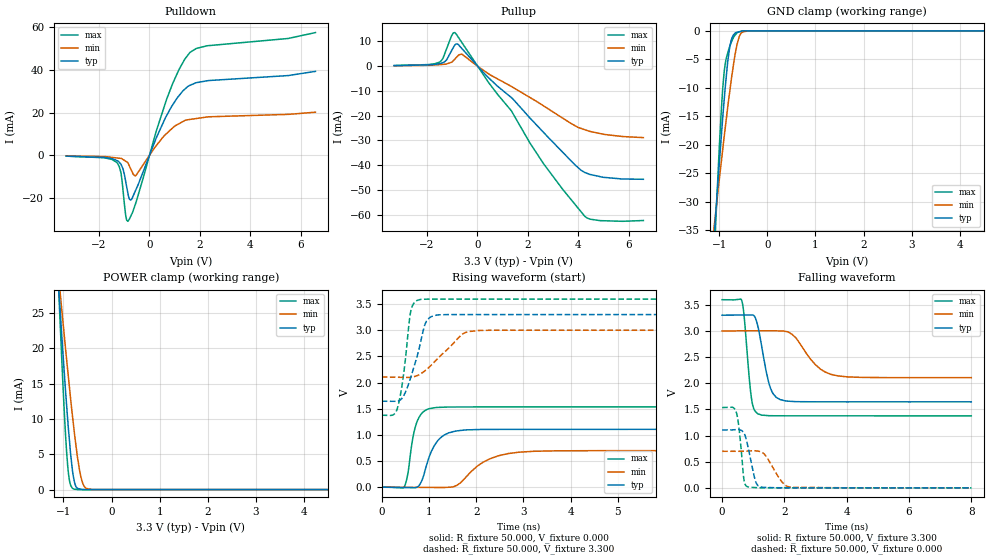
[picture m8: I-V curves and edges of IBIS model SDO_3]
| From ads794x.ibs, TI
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|   SDO 3.3V Model
[Model] SDO_3
Model_type   3-state
Polarity   Non-Inverting
Enable   Active-Low
Vmeas = 1.65
Vref = 1.65
Cref = 15pF
Rref = 50
|   typ   min   max
|   (Nom PVT)   (Fast PVT)  (Slow PVT)
|  (high input impedance)
C_comp   1.5797330e-12   1.2761490e-12   1.9045100e-12
|  (high output)
|C_comp   2.1280980e-12   1.7654750e-12   2.4622910e-12
|  (low output)
|C_comp   1.0558410e-12   8.2578200e-13   1.4524100e-12
[Voltage Range]   3.3   3   3.6
[Temperature Range]   27   125   -40
[Pullup Reference]   3.3   3   3.6
[Pulldown Reference]   0   0   0
[Power Clamp Reference]   3.3   3   3.6
[GND Clamp Reference]   0   0   0
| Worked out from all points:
|   slope of the pulldown table from 0 to 0.495 V, typ, clamps not added: 35.2 ohm
|   slope of the pullup table from 0 to 0.495 V, typ, clamps not added: 93 ohm
|   GND clamp passes 1 mA (typ) near -0.72 V on its own axis
|   POWER clamp passes 1 mA (typ) near -0.77 V on its own axis
|   falling waveform, R_fixture 50.000, V_fixture 3.300: 20-80 % time 325ps typ, 704ps min, 192ps max; typ from 3.3 V to 1.64 V
|   rising waveform, R_fixture 50.000, V_fixture 0.000: 20-80 % time 296ps typ, 612ps min, 176ps max; typ from 0 V to 1.11 V
|   rising waveform, R_fixture 50.000, V_fixture 3.300: 20-80 % time 302ps typ, 595ps min, 174ps max; typ from 1.64 V to 3.3 V
|   falling waveform, R_fixture 50.000, V_fixture 0.000: 20-80 % time 238ps typ, 426ps min, 149ps max; typ from 1.11 V to 0 V
[Pulldown]
|   Voltage   I(typ)   I(min)   I(max)
-3.3V     -352.2uA   -233.3uA   -375.8uA
-1.293V   -2.417mA   -1.214mA   -3.331mA
-1.135V   -4.022mA   -1.435mA   -7.896mA
-947mV    -11.94mA   -2.7mA     -27.63mA
-859.1mV  -17.48mA   -3.397mA   -30.89mA
-747.5mV  -20.98mA   -6.21mA    -28.68mA
-544.8mV  -16.32mA   -9.497mA   -22.46mA
688.3mV   18.76mA    10.3mA     26.47mA
1.169V    27.89mA    14.8mA     40.07mA
1.596V    32.73mA    16.8mA     48.04mA
2.285V    34.93mA    17.97mA    51.32mA
6.59V     39.34mA    20.22mA    57.52mA
[GND Clamp]
|   Voltage   I(typ)   I(min)   I(max)
-3.3V     -328.8mA   -220.3mA   -502.7mA
-1.091V   -34.15mA   -33.2mA    -37.08mA
-1.069V   -31.46mA   -31.46mA   -32.81mA
-962.1mV  -19.04mA   -23.34mA   -14.63mA
-925.9mV  -15mA      -20.65mA   -9.896mA
-894.4mV  -11.8mA    -18.35mA   -6.959mA
-790mV    -3.26mA    -11.15mA   -2.902mA
-733mV    -1.183mA   -7.554mA   -1.68mA
-658.6mV  -306.6uA   -3.608mA   -629.6uA
-552.4mV  -101.2uA   -492.2uA   -91.33uA
-387.7mV  -8.397uA   -5.302uA   -27.14uA
6.59V     0A         0A         0A
[Pullup]
|   Voltage   I(typ)   I(min)   I(max)
-3.3V     186uA      133.8uA    217.3uA
-1.51V    980uA      572.5uA    1.547mA
-1.223V   2.485mA    849.4uA    6.91mA
-1.022V   6.221mA    1.561mA    12.26mA
-894.4mV  8.451mA    2.812mA    13.54mA
-602.7mV  6.957mA    4.705mA    9.331mA
437mV     -4.631mA   -3.064mA   -6.524mA
1.346V    -12.7mA    -8.209mA   -18.02mA
2.658V    -27.13mA   -16.28mA   -39.88mA
4.258V    -42.95mA   -25.69mA   -60.62mA
4.872V    -44.67mA   -27.26mA   -62.45mA
6.59V     -45.74mA   -28.9mA    -62.4mA
[POWER Clamp]
|   Voltage   I(typ)   I(min)   I(max)
-3.3V     294.5mA    213.9mA    419.3mA
-1.091V   27.74mA    29.53mA    27.09mA
-1.06V    24.48mA    27.26mA    22.29mA
-970.1mV  15.31mA    20.9mA     9.4mA
-911.7mV  9.92mA     16.9mA     3.379mA
-859.1mV  5.671mA    13.4mA     812.3uA
-778.4mV  1.317mA    8.386mA    59.57uA
-708.3mV  165.6uA    4.588mA    5.929uA
-612mV    12.27uA    1.17mA     5.098uA
-530.5mV  3.607uA    177.8uA    5.04uA
-404.5mV  3.544uA    4.964uA    4.951uA
6.59V     0A         0A         0A
[Ramp]
R_load = 50
|   typ   min   max
dV/dt_r   0.664025/2.95396e-010  0.419237/6.00764e-010  0.921081/1.75378e-010
dV/dt_f   0.99364/3.23576e-010  0.535755/6.98515e-010   1.39626/1.91318e-010
[Falling Waveform]
R_fixture = 50.000
V_fixture = 3.300
V_fixture_min = 3.000
V_fixture_max = 3.600
C_fixture = 0.000
|  time   V(typ)   V(min)   V(max)
0s        3.3V       3V         3.596V
628ps     3.303V     3.001V     3.585V
708.5ps   3.303V     3.001V     3.273V
938.4ps   3.304V     3.001V     1.727V
1.146ns   3.093V     3.001V     1.416V
1.515ns   1.975V     3.001V     1.379V
1.862ns   1.687V     2.999V     1.378V
2.246ns   1.652V     2.935V     1.377V
3.515ns   1.644V     2.166V     1.377V
8ns       1.644V     2.107V     1.376V
[Rising Waveform]
R_fixture = 50.000
V_fixture = 0.000
V_fixture_min = 0.000
V_fixture_max = 0.000
C_fixture = 0.000
|  time   V(typ)   V(min)   V(max)
0s        5.249uV    20.61uV    1.893uV
475.1ps   -6.977mV   -2.25mV    2.15mV
555.5ps   -8.157mV   -2.634mV   269.2mV
731ps     -3.975mV   -3.472mV   1.21V
838.4ps   104.9mV    -3.986mV   1.401V
1.008ns   586.4mV    -4.797mV   1.502V
1.418ns   1.039V     -1.039mV   1.533V
2.274ns   1.105V     536.6mV    1.535V
2.903ns   1.106V     668.8mV    1.535V
8ns       1.107V     698.7mV    1.535V
[Rising Waveform]
R_fixture = 50.000
V_fixture = 3.300
V_fixture_min = 3.000
V_fixture_max = 3.600
C_fixture = 0.000
|  time   V(typ)   V(min)   V(max)
0s        1.644V     2.107V     1.376V
327.2ps   1.641V     2.102V     1.496V
461.3ps   1.744V     2.1V       2.147V
613.4ps   2.095V     2.103V     3.358V
748.5ps   2.498V     2.133V     3.572V
928.5ps   3.141V     2.236V     3.594V
1.195ns   3.295V     2.468V     3.596V
1.707ns   3.301V     2.926V     3.596V
2.038ns   3.301V     2.996V     3.596V
8ns       3.3V       3V         3.596V
[Falling Waveform]
R_fixture = 50.000
V_fixture = 0.000
V_fixture_min = 0.000
V_fixture_max = 0.000
C_fixture = 0.000
|  time   V(typ)   V(min)   V(max)
0s        1.107V     698.7mV    1.535V
331.1ps   1.108V     698.8mV    1.542V
453.5ps   1.113V     698.8mV    1.449V
556.4ps   1.112V     698.8mV    1.065V
691.5ps   1.057V     700.7mV    198.3mV
810.6ps   839.4mV    703.7mV    21.97mV
1.078ns   116.9mV    707.1mV    5.386mV
1.224ns   19.68mV    690.7mV    2.102mV
2.146ns   1.277mV    18.66mV    269.5uV
8ns       5.249uV    20.61uV    1.893uV
